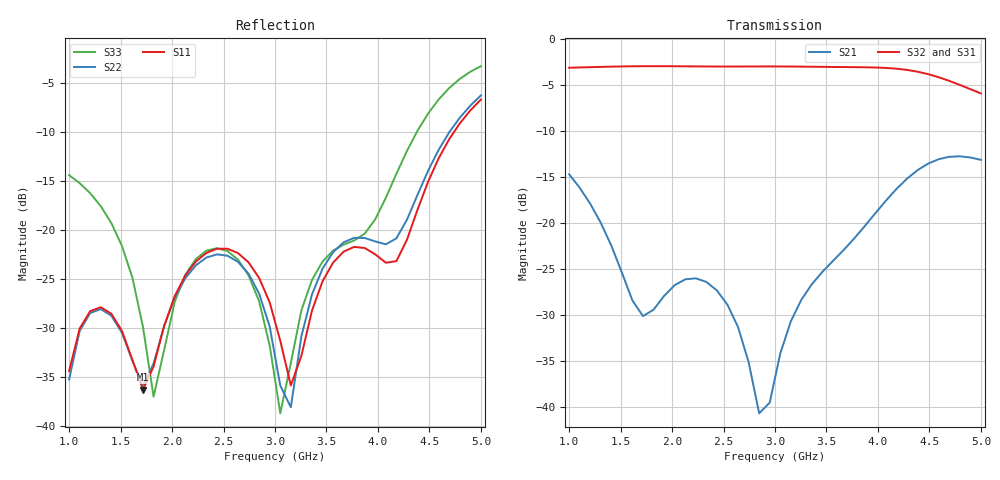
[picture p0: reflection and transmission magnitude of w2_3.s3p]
# GHZ S RI R 50
!Output file by EM3DS 5.12 Built 1
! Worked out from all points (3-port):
!   40 points, 1 GHz to 5 GHz, reference 50 ohm
!   strongest paths, dB at 1 GHz, 2.026 GHz, 3.051 GHz, 4.077 GHz, 5 GHz:
!     S32: -3.2, -3.0, -3.0, -3.2, -5.9
!     S31: -3.2, -3.1, -3.1, -3.2, -5.9
!     S21: -14.7, -26.7, -34.1, -17.6, -13.2
!   lowest |S11| = -36.3 dB at 1.718 GHz (marker M1), VSWR 1.03, Z = 49.1 + j1.24 ohm
!   |S11| at or under -10 dB: start of sweep to 4.739 GHz
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1  -0.00835 0.0172  -0.1733 -0.0612  -0.4191 -0.5521
   -0.1733 -0.0612  -0.0142 0.00982  -0.4214 -0.5522
   -0.4191 -0.5521  -0.4214 -0.5522  -0.0025 0.1905
1.307692  -0.0105 0.039  -0.087 0.0497  -0.6658 -0.2125
          -0.087 0.0497  -0.016 0.0361  -0.6697 -0.2101
          -0.6658 -0.2125  -0.6697 -0.2101  0.0321 0.1283
1.717949  -0.00862 0.0127  0.0277 0.0144  -0.6048 0.3598
          0.0277 0.0144  -0.0105 0.0121  -0.6057 0.3666
          -0.6048 0.3598  -0.6057 0.3666  0.0142 0.0286
1.820513  -0.019 0.00668  0.0328 -0.0084  -0.5144 0.4803
          0.0328 -0.0084  -0.02 0.00607  -0.5137 0.4876
          -0.5144 0.4803  -0.5137 0.4876  -0.00381 0.0136
2.435897  -0.0515 0.0616  -0.0273 -0.0333  0.3192 0.6237
          -0.0273 -0.0333  -0.0486 0.0573  0.3284 0.624
          0.3192 0.6237  0.3284 0.624  -0.0644 0.0488
2.846154  -0.000428 0.0569  -0.00607 -0.00704  0.6841 0.1568
          -0.00607 -0.00704  0.00028 0.0473  0.6899 0.1485
          0.6841 0.1568  0.6899 0.1485  -0.0133 0.0411
3.051282  0.00161 0.0272  0.0102 -0.0168  0.6857 -0.1515
          0.0102 -0.0168  -0.000953 0.0161  0.6868 -0.1619
          0.6857 -0.1515  0.6868 -0.1619  -0.00945 0.00675
3.666667  -0.0697 0.0341  0.00503 -0.0712  0.00142 -0.6988
          0.00503 -0.0712  -0.0824 0.0266  -0.0101 -0.7003
          0.00142 -0.6988  -0.0101 -0.7003  -0.0695 0.0476
4.179487  -0.0645 0.0256  -0.074 -0.1337  -0.6361 -0.2583
          -0.074 -0.1337  -0.0861 0.0285  -0.6407 -0.2461
          -0.6361 -0.2583  -0.6407 -0.2461  0.1931 0.0151
5  -0.2126 0.4112  -0.1937 0.1041  -0.0326 0.5083
   -0.1937 0.1041  -0.1985 0.4435  -0.0203 0.5038
   -0.0326 0.5083  -0.0203 0.5038  -0.3749 -0.5736
